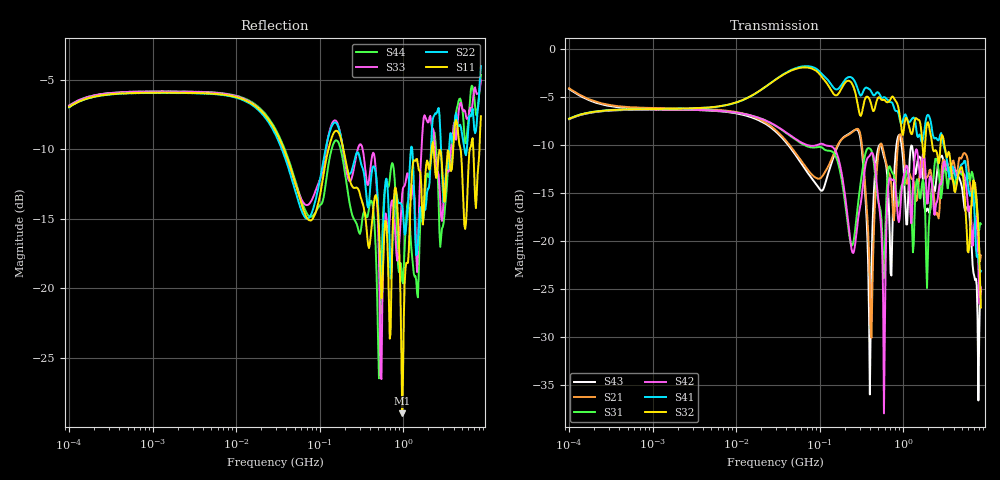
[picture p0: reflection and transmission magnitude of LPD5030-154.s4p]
# MHz S MA R 50
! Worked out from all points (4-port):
!   498 points, 100 kHz to 8.5 GHz, reference 50 ohm
!   strongest paths, dB at 100 kHz, 1.698 MHz, 29.49 MHz, 500.7 MHz, 8.5 GHz:
!     S32: -7.3, -6.3, -3.2, -5.1, -27.0
!     S41: -7.3, -6.3, -3.2, -4.5, -23.2
!     S42: -7.3, -6.3, -8.0, -15.6, -24.9
!     S31: -7.3, -6.3, -8.0, -15.9, -18.3
!     S21: -4.1, -6.2, -8.4, -11.2, -21.6
!     S43: -4.2, -6.3, -8.6, -10.4, -25.3
!   lowest |S11| = -29.0 dB at 970.9 MHz (marker M1), VSWR 1.07, Z = 47.5 - j2.36 ohm
!   |S11| at or under -10 dB: 192 MHz to 2.192 GHz (2 GHz wide, 168 % of centre); 2.315 GHz to 3.965 GHz (1.649 GHz wide, 52.5 % of centre); 4.842 GHz to 6.278 GHz (1.436 GHz wide, 25.8 % of centre)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
0.1  0.448 25.5  0.6228 -18.5  0.4299 -153.3  0.4324 27.0
     0.6228 -18.5  0.4463 25.5  0.4315 27.0  0.43 -153.4
     0.4299 -153.3  0.4315 27.0  0.4534 25.5  0.618 -18.8
     0.4324 27.0  0.43 -153.4  0.618 -18.8  0.4535 25.6
68.6511  0.1813 -27.2  0.2403 -106.4  0.3119 73.5  0.8118 -10.0
         0.2403 -106.4  0.1781 -17.3  0.7996 -12.5  0.3165 71.9
         0.3119 73.5  0.7996 -12.5  0.1992 -17.3  0.2322 -109.3
         0.8118 -10.0  0.3165 71.9  0.2322 -109.3  0.188 -30.9
289.4033  0.227 -63.0  0.3813 -7.9  0.1596 102.1  0.6064 -56.6
          0.3813 -7.9  0.3069 -51.1  0.4939 -62.8  0.1317 95.0
          0.1596 102.1  0.4939 -62.8  0.3203 -42.7  0.3736 -15.0
          0.6064 -56.6  0.1317 95.0  0.3736 -15.0  0.1623 -55.0
398.4376  0.1445 -62.6  0.05826 -70.1  0.3018 -4.4  0.6131 -69.1
          0.05826 -70.1  0.2213 -54.7  0.5406 -69.4  0.2784 -4.5
          0.3018 -4.4  0.5406 -69.4  0.259 -62.1  0.01579 -27.3
          0.6131 -69.1  0.2784 -4.5  0.01579 -27.3  0.2017 -61.6
970.9031  0.03551 -135.7  0.3358 -119.3  0.1955 -104.3  0.4128 -145.3
          0.3358 -119.3  0.1973 -127.8  0.3629 -156.3  0.1945 -82.2
          0.1955 -104.3  0.3629 -156.3  0.218 -97.6  0.2966 -127.7
          0.4128 -145.3  0.1945 -82.2  0.2966 -127.7  0.1062 -132.1
7244.201  0.2104 153.9  0.2 136.4  0.1802 123.7  0.119 103.3
          0.2 136.4  0.3606 175.1  0.1892 92.1  0.1296 128.3
          0.1802 123.7  0.1892 92.1  0.527 -170.5  0.06226 138.6
          0.119 103.3  0.1296 128.3  0.06226 138.6  0.4505 171.0
8500  0.415 -27.0  0.08364 -21.0  0.1222 -19.0  0.0695 -12.4
      0.08364 -21.0  0.6282 -26.1  0.04486 176.5  0.05711 -3.6
      0.1222 -19.0  0.04486 176.5  0.5591 -12.4  0.05449 52.1
      0.0695 -12.4  0.05711 -3.6  0.05449 52.1  0.5842 -22.9
